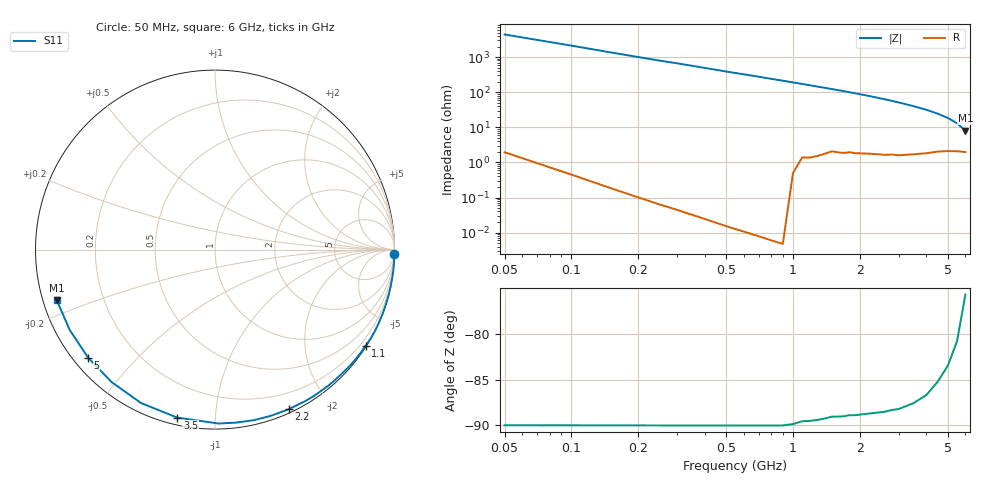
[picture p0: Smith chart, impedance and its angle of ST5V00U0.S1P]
! SIEMENS Discrete & RF Semiconductors
! BA892
! Si PIN Diode in SCD-80
! VR = 5 V
! S-Parameters:  September  1997
# GHz  S  MA  R  50
!  f  S11
! GHz  MAG  ANG
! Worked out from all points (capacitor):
!   34 points, 50 MHz to 6 GHz, reference 50 ohm
!   read as one part to ground: C = 750 fF near 50 MHz
!   lowest |Z| = 8.02 ohm at 6 GHz (marker M1)
!   S11 on the Smith chart (normalised r, x): 50 MHz: 0, -88; 1.1 GHz: 0.03, -3.43; 2.2 GHz: 0.04, -1.56; 3.5 GHz: 0.03, -0.80; 5 GHz: 0.04, -0.37; 6 GHz: 0.04, -0.16
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0.05  1 -1.3
0.2  1 -5.7
0.4  1 -11.6
0.5  1 -14.7
0.6  1 -17.6
0.7  1 -20.5
0.8  1 -23.6
0.9  1 -26.5
1  0.9987 -29.5
1.1  0.9957 -32.5
1.2  0.9949 -35.4
1.3  0.9933 -38.5
1.4  0.9911 -41.4
1.6  0.9876 -47.3
1.7  0.9866 -50.3
1.9  0.9839 -56.2
2  0.9824 -59.2
2.2  0.9796 -65.2
2.4  0.9771 -71.2
2.6  0.9748 -77.1
2.8  0.9711 -83.0
3  0.9692 -88.8
3.5  0.9594 -102.6
4  0.949 -115.7
4.5  0.9364 -128.0
5  0.9286 -139.6
5.5  0.9249 -151.1
6  0.9256 -162.3
